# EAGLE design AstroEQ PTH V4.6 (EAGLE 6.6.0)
REVISION: V4.6
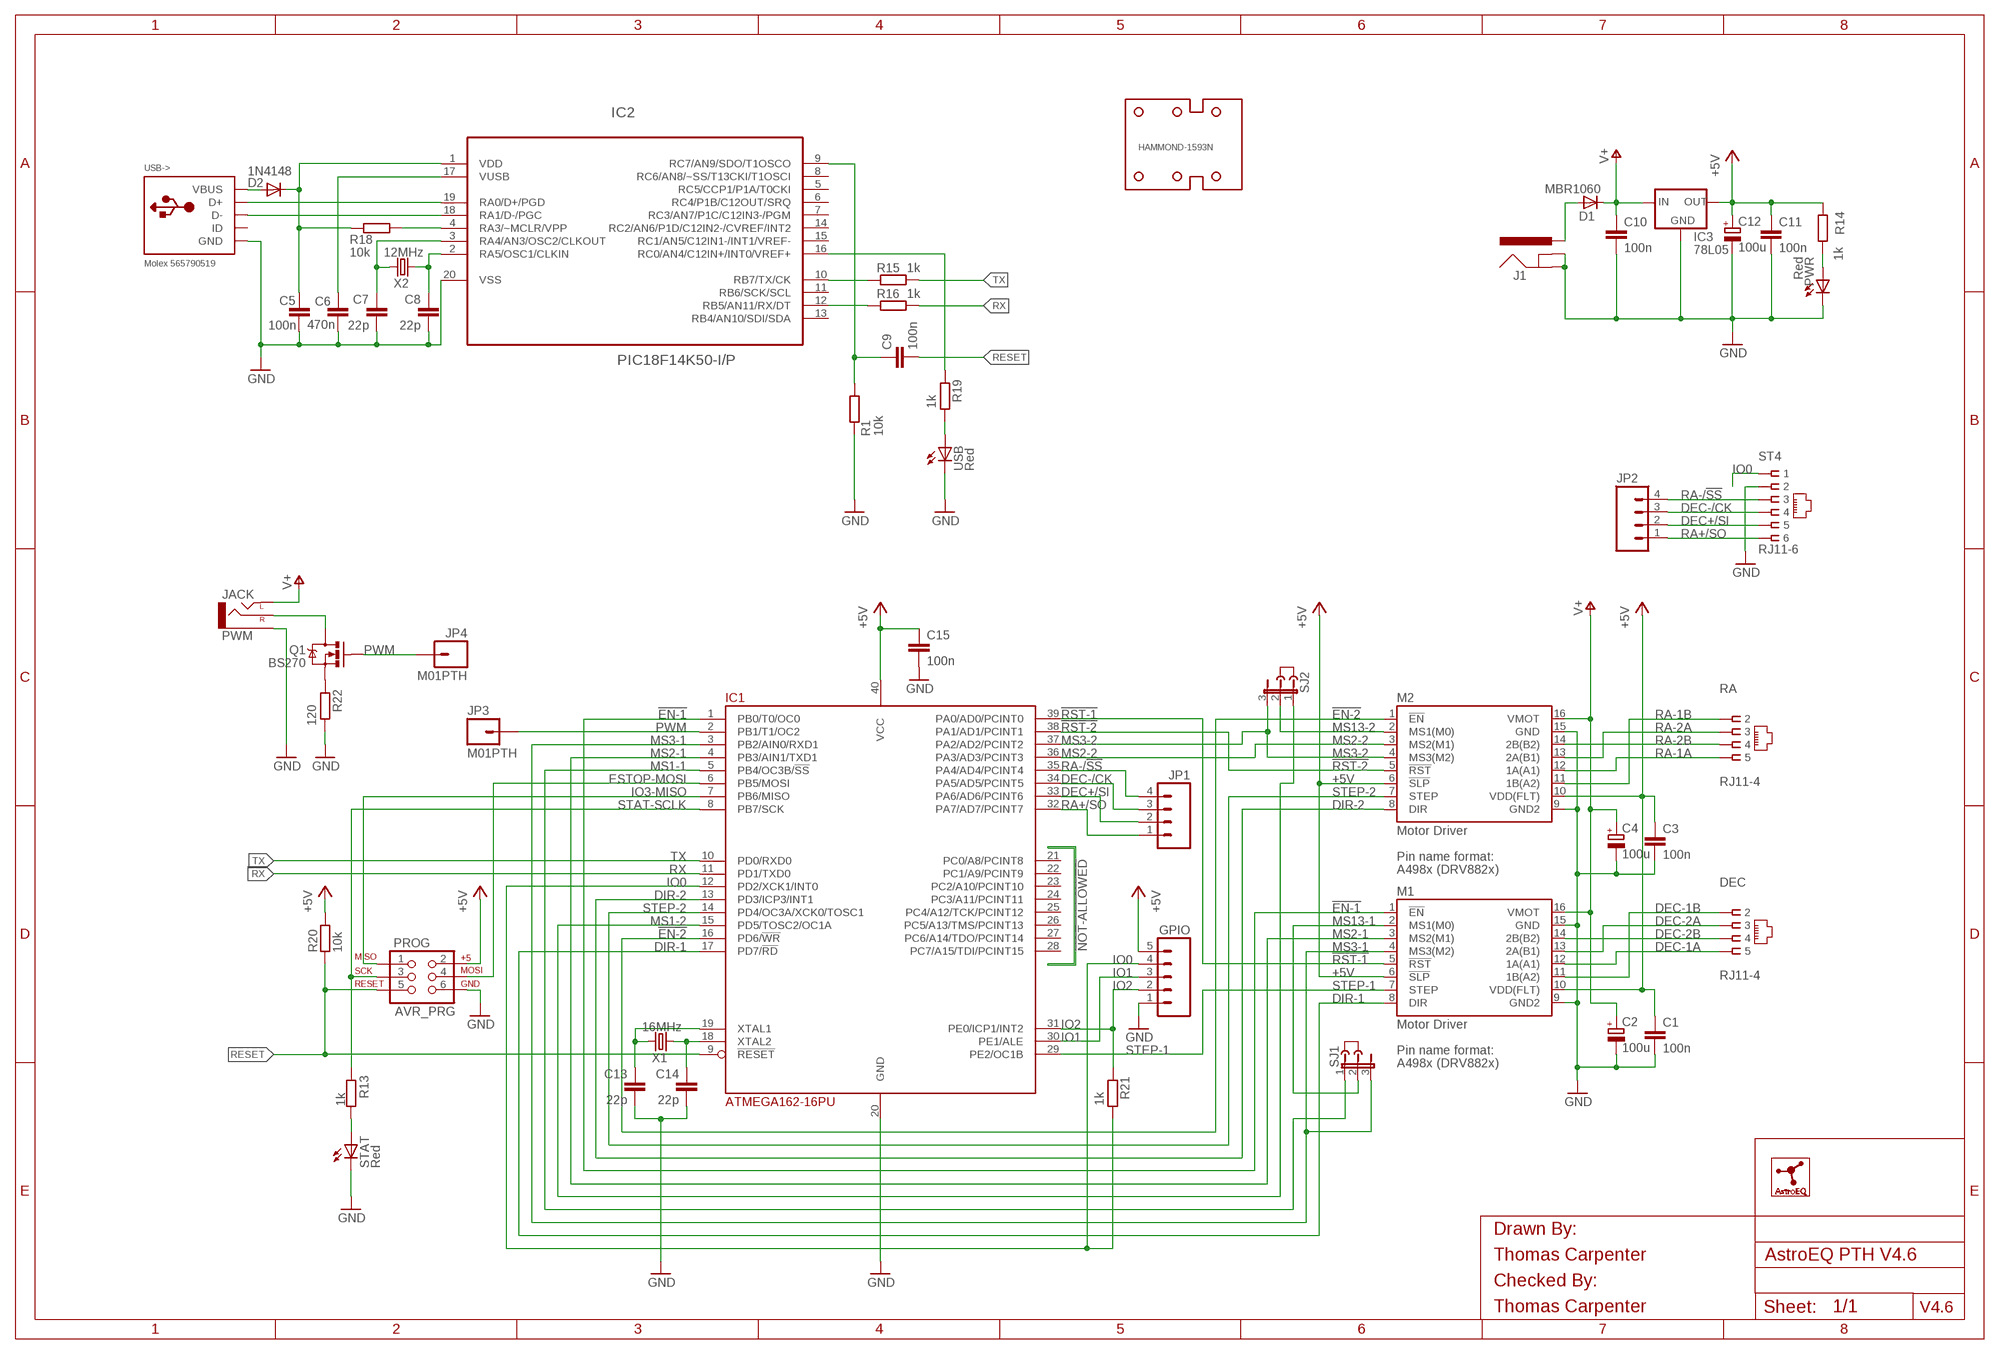
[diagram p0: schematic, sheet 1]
FRAME1 (A3L-LOC): CHECKED_BY: Thomas Carpenter; DRAWN_BY: Thomas Carpenter

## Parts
C1  100n  C-EU025-024X044  [C025-024X044]
C2  100u  CPOL-EUE2.5-7  [E2,5-7]
C3  100n  C-EU025-024X044  [C025-024X044]
C4  100u  CPOL-EUE2.5-7  [E2,5-7]
C5  100n  C-EU025-024X044  [C025-024X044]
C6  470n  C-EU025-024X044  [C025-024X044]
C7  22p  C-EU025-024X044  [C025-024X044]
C8  22p  C-EU025-024X044  [C025-024X044]
C9  100n  C-EU025-024X044  [C025-024X044]
C10  100n  C-EU025-024X044  [C025-024X044]
C11  100n  C-EU025-024X044  [C025-024X044]
C12  100u  CPOL-EUE2.5-7  [E2,5-7]
C13  22p  C-EU025-024X044  [C025-024X044]
C14  22p  C-EU025-024X044  [C025-024X044]
C15  100n  C-EU025-024X044  [C025-024X044]
D1  MBR1060  MUR820  [C221B1A]
D2  1N4148  DIODE1N4148  [DIODE-1N4148]
DEC  RJ11-4  [RJ11-NO_SHIELD-4]
GPIO  M05PTH  [1X05]
HAMMOND-1593N  HAMMOND-1593N-4HOLE  [HAMMOND-1593N4HOLES]
IC1  ATMEGA162-16PU  [DIL40]
IC2  PIC18F14K50-I/P  [DIL20]
IC3  78L05  V_REG_78XXTO-92  [TO-92]
J1  POWER_JACKPTH  [POWER_JACK_PTH]
J2  JUMPER  [JUMP]
J3  JUMPER  [JUMP]
JP1  M04PTH  [1X04]
JP2  M04PTH  [1X04]
JP3  M01PTH  [1X01]
JP4  M01PTH  [1X01]
LOGO1  ASTROEQ5MM  [ASTROEQ-SMALL]
M1  Motor Driver  A4983CARRIER  [DIP16-W]
M2  Motor Driver  A4983CARRIER  [DIP16-W]
PROG  AVR_PRG  AVR_SPI_PRG_6PTH  [2X3]
PWM  JACK  AUDIO-JACKPTH  [AUDIO-JACK]
PWR  Red  LED3MM  [LED3MM]
Q1  BS270  MOSFET-NCHANNELPTH  [TO-92]
R1  10k  R-EU_0204/7  [0204/7]
R13  1k  R-EU_0204/7  [0204/7]
R14  1k  R-EU_0204/7  [0204/7]
R15  1k  R-EU_0204/7  [0204/7]
R16  1k  R-EU_0204/7  [0204/7]
R18  10k  R-EU_0204/7  [0204/7]
R19  1k  R-EU_0204/7  [0204/7]
R20  10k  R-EU_0204/7  [0204/7]
R21  1k  R-EU_0204/7  [0204/7]
R22  120  R-EU_0204/7  [0204/7]
RA  RJ11-4  [RJ11-NO_SHIELD-4]
SJ1  JP2E  [JP2]
SJ2  JP2EL  [JP2L]
ST4  RJ11-6  RJ11-2L-B  [RJ11-NO_SHIELD]
STAT  Red  LED3MM  [LED3MM]
USB  Red  LED3MM  [LED3MM]
USB->  Molex 565790519  USBMOLEX  [USB-MINIB-THM-MOLEX]
X1  16MHz  CRYSTALHC49US  [HC49US]
X2  12MHz  CRYSTALHC49US  [HC49US]

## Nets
!EN-1: IC1.1(PB0/T0/OC0) M1.1(!EN)
!EN-2: IC1.16(PD6/!WR) M2.1(!EN)
!RST-1: IC1.39(PA0/AD0/PCINT0) M1.5(!RST)
!RST-2: IC1.38(PA1/AD1/PCINT1) M2.5(!RST)
+5V: C1.1 C3.1 C11.1 C12.+ C15.1 GPIO.5 IC1.40(VCC) IC3.1(OUT) M1.6(!SLP) M1.10(VDD(FLT)) M2.6(!SLP) M2.10(VDD(FLT)) PROG.2 R14.1 R20.2
AVROSC1: C13.1 IC1.19(XTAL1) X1.2
AVROSC2: C14.1 IC1.18(XTAL2) X1.1
D+: IC2.19(RA0/D+/PGD) USB->.D+
D-: IC2.18(RA1/D-/PGC) USB->.D-
DEC+/SI: IC1.33(PA6/AD6/PCINT6) JP1.2 JP2.2 ST4.5
DEC-1A: DEC.5 M1.12(1A(A1))
DEC-1B: DEC.2 M1.11(1B(A2))
DEC-2A: DEC.3 M1.13(2A(B1))
DEC-2B: DEC.4 M1.14(2B(B2))
DEC-/CK: IC1.34(PA5/AD5/PCINT5) JP1.3 JP2.3 ST4.4
DIR-1: IC1.17(PD7/!RD) M1.8(DIR)
DIR-2: IC1.13(PD3/ICP3/INT1) M2.8(DIR)
DTR: C9.1 IC2.9(RC7/AN9/SDO/T1OSCO) R1.1
ESTOP-MOSI: IC1.6(PB5/MOSI) PROG.4
GND: C1.2 C2.- C3.2 C4.- C5.2 C6.1 C7.2 C8.2 C10.2 C11.2 C12.- C13.2 C14.2 C15.2 GPIO.1 IC1.20(GND) IC2.20(VSS) IC3.2(GND) J1.GND J1.GNDBREAK M1.9(GND2) M1.15(GND) M2.9(GND2) M2.15(GND) PROG.6 PWM.SLEEVE PWR.K(C) R1.2 R22.1 ST4.2 STAT.K(C) USB->.GND USB->.GND1(GND) USB->.GND4(GND) USB.K(C)
IO0: GPIO.4 IC1.12(PD2/XCK1/INT0) R21.1 ST4.1
IO1: GPIO.3 IC1.30(PE1/ALE)
IO2: GPIO.2 IC1.31(PE0/ICP1/INT2) R21.2
IO3-MISO: IC1.7(PB6/MISO) PROG.1
MCLR: IC2.4(RA3/~MCLR/VPP) R18.1
MS1-1: IC1.5(PB4/OC3B/!SS) SJ1.1
MS1-2: IC1.15(PD5/TOSC2/OC1A) SJ2.1
MS2-1: IC1.4(PB3/AIN1/TXD1) M1.3(MS2(M1))
MS2-2: IC1.36(PA3/AD3/PCINT3) M2.3(MS2(M1))
MS3-1: IC1.3(PB2/AIN0/RXD1) M1.4(MS3(M2)) SJ1.3
MS3-2: IC1.37(PA2/AD2/PCINT2) M2.4(MS3(M2)) SJ2.3
MS13-1: M1.2(MS1(M0)) SJ1.2
MS13-2: M2.2(MS1(M0)) SJ2.2
PWM: IC1.2(PB1/T1/OC2) JP3.1 JP4.1 Q1.2(G)
PWM-ILIM: Q1.3(S) R22.2
PWM-OUT: PWM.RING(RIGHT) Q1.1(D)
PWRLED: PWR.A R14.2
RA+/SO: IC1.32(PA7/AD7/PCINT7) JP1.1 JP2.1 ST4.6
RA-1A: M2.12(1A(A1)) RA.5
RA-1B: M2.11(1B(A2)) RA.2
RA-2A: M2.13(2A(B1)) RA.3
RA-2B: M2.14(2B(B2)) RA.4
RA-/!SS: IC1.35(PA4/AD4/PCINT4) JP1.4 JP2.4 ST4.3
RESET: C9.2 IC1.9(!RESET) PROG.5 R20.1
RX: IC1.11(PD1/TXD0) R16.1
RX(USB): IC2.12(RB5/AN11/RX/DT) R16.2
STAT-SCLK: IC1.8(PB7/SCK) PROG.3 R13.1
STATLED: R13.2 STAT.A
STEP-1: IC1.29(PE2/OC1B) M1.7(STEP)
STEP-2: IC1.14(PD4/OC3A/XCK0/TOSC1) M2.7(STEP)
TX: IC1.10(PD0/RXD0) R15.1
TX(USB): IC2.10(RB7/TX/CK) R15.2
USBLED: R19.1 USB.A
USBOSC1: C8.1 IC2.2(RA5/OSC1/CLKIN) X2.1
USBOSC2: C7.1 IC2.3(RA4/AN3/OSC2/CLKOUT) X2.2
USBSTAT: IC2.16(RC0/AN4/C12IN+/INT0/VREF+) R19.2
V+: C2.+ C4.+ C10.1 D1.C IC3.3(IN) M1.16(VMOT) M2.16(VMOT) PWM.TIP(LEFT)
VBUS: D2.A USB->.VBUS
VIN: D1.A J1.PWR
VPIC: C5.1 D2.C IC2.1(VDD) R18.2
VUSB: C6.2 IC2.17(VUSB)
Unconnected: IC1.21(PC0/A8/PCINT8) IC1.22(PC1/A9/PCINT9) IC1.23(PC2/A10/PCINT10) IC1.24(PC3/A11/PCINT11) IC1.25(PC4/A12/TCK/PCINT12) IC1.26(PC5/A13/TMS/PCINT13) IC1.27(PC6/A14/TDO/PCINT14) IC1.28(PC7/A15/TDI/PCINT15) IC2.5(RC5/CCP1/P1A/T0CKI) IC2.6(RC4/P1B/C12OUT/SRQ) IC2.7(RC3/AN7/P1C/C12IN3-/PGM) IC2.8(RC6/AN8/~SS/T13CKI/T1OSCI) IC2.11(RB6/SCK/SCL) IC2.13(RB4/AN10/SDI/SDA) IC2.14(RC2/AN6/P1D/C12IN2-/CVREF/INT2) IC2.15(RC1/AN5/C12IN1-/INT1/VREF-) USB->.ID

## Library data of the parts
C1 C3 C5 C9-C11 C15 = resistor:C-EU: CAPACITOR, European symbol; MF: AVX; MPN: SR205C104KAR; OC_FARNELL: 1100367
C2 C4 C12 = resistor:CPOL-EU: POLARIZED CAPACITOR, European symbol; MF: MULTICOMP; MPN: MCGPR25V107M6.3X11; OC_FARNELL: 9451188
C6 = resistor:C-EU: CAPACITOR, European symbol; MF: KEMET; MPN: C320C474M5U5TA; OC_FARNELL: 1457660
C7 C8 C13 C14 = resistor:C-EU: CAPACITOR, European symbol; MF: AVX; MPN: SR151A220JAR; OC_FARNELL: 1100369
D1 = diode:MUR820: DIODE; MF: MULTICOMP; MPN: MBR1060; OC_FARNELL: 1625119
D2 = SparkFun:DIODE: Diode; MF: MULTICOMP; MPN: 1N4148.; OC_FARNELL: 9565124
DEC RA = con-tycoelectronics:RJ11-4; MF: MOLEX; MPN: 95501-2641; OC_FARNELL: 1560166
GPIO = SparkFun:M05: Header 5 Standard 5-pin 0.1" header. Use with straight break away headers (SKU : PRT-00116), right angle break away headers (PRT-00553), swiss pins (PRT-00743), machine pins (PRT-00117), and female headers (PRT-00115). Molex polarized connector foot print use with SKU : PRT-08230 with associated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; MF: CYNERGY3; MPN: SSF211X050; OC_FARNELL: 4249100
HAMMOND-1593N = holes:HAMMOND-1593N; MF: HAMMOND; MPN: 1593NBK; OC_FARNELL: 9287566
IC1 = atmel:ATMEGA162: 8-bit RISC MICROCONTROLLER 16K Bytes internal flash program memory 1K Bytes internal SRAM Upto 64K Bytes optional external memory space 512 Bytes EEPROM Two 8-bit timers Two 16-bit timers Dual programmable serial USARTs Master/Slave serial SPI interface Source: ATMEGA162_DIP40.lbr; MF: ATMEL; MPN: ATMEGA162-16PU; OC_FARNELL: 9171169
IC2 = microchip:PIC18F14K50-I/P: USB Flash Microcontrollers; MF: MICROCHIP; MPN: PIC18F14K50-I/P; OC_FARNELL: 1648501; OC_NEWARK: 77M3103; PACKAGE: DIP-20; SUPPLIER: Microchip
IC3 = SparkFun:V_REG_78XX: Voltage Regulator Standard 7805 5V regulator. IGO (Input Ground Output). Spark Fun Electronics SKU : COM-00107; MF: FAIRCHILD SEMICONDUCTOR; MPN: LM78L05ACZX; OC_FARNELL: 1467367
J1 = SparkFun:POWER_JACK: Power Jack This is the standard 5.5mm barrel jack for power. The PTH is the most common, proven, reliable, footprint. All others are experimental. The Slot footprint only works if the mill layer is transmitted to the PCB fab house so be warned. Spark Fun Electronics SKU : PRT-00119. Mating wall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; MF: MULTICOMP; MPN: MJ-179PH; OC_FARNELL: 1737246
J2 J3 = jumper:JUMPER: JUMPER header; OC_FARNELL: unknown
JP1 JP2 = SparkFun:M04: Header 4 Standard 4-pin 0.1" header. Use with straight break away headers (SKU : PRT-00116), right angle break away headers (PRT-00553), swiss pins (PRT-00743), machine pins (PRT-00117), and female headers (PRT-00115). Molex polarized connector foot print use with SKU : PRT-08231 with associated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; OC_FARNELL: unknown
JP3 JP4 = SparkFun:M01: Header 1; OC_FARNELL: unknown
LOGO1 = CompanyLogos:ASTROEQ; OC_FARNELL: unknown
M1 M2 = A4983Carrier:A4983CARRIER; MF: SAMTEC; MPN: CES-116-01-T-S; OC_FARNELL: 1667522
PROG = SparkFun:AVR_SPI_PRG_6: AVR ISP 6 Pin This is the reduced ISP connector for AVR programming. Common on Arduino. This footprint will take up less PCB space and can be used with a 10-pin to 6-pin adapter such as SKU: BOB-08508; MF: TE CONNECTIVITY / AMP; MPN: 826632-3; OC_FARNELL: 3418492
PWM = SparkFun:AUDIO-JACK: 3.5mm Audio Jack Simple 3.5mm common PCB mount audio jack. SKU: PRT-08032; MF: CLIFF ELECTRONIC COMPONENTS; MPN: FC68131; OC_FARNELL: 2518188
PWR STAT USB = led:LED: LED; MF: KINGBRIGHT; MPN: L-424HDT; OC_FARNELL: 1142499
Q1 = SparkFun:MOSFET-NCHANNEL; MF: FAIRCHILD SEMICONDUCTOR; MPN: BS270; OC_FARNELL: 1017689
R1 R18 R20 = rcl:R-EU_: RESISTOR, European symbol; MF: MULTICOMP; MPN: MF12 10K; OC_FARNELL: 9342419
R13-R16 R19 R21 = rcl:R-EU_: RESISTOR, European symbol; MF: MULTICOMP; MPN: MF12 1K; OC_FARNELL: 9342400
R22 = rcl:R-EU_: RESISTOR, European symbol; MF: MULTICOMP; MPN: MF12 120R; OC_FARNELL: 9342516
SJ1 SJ2 = jumper:JP2E: JUMPER; OC_FARNELL: unknown
ST4 = con-tycoelectronics:RJ11: CORCOM Modular RJ Jacks No Shield Source: www.tycoelectronics.com .. ENG_DS_1654001_1099_RJ_L_0507.pdf; MF: MOLEX; MPN: 95501-2661; OC_FARNELL: 1536490; OC_NEWARK: 83F4463
USB-> = adafruit:USB: USB Connectors USBMINIB - Surface Mount Female Mini-B USB Connector 4UConnector: 06564 By microbuilder.eu Thru-hole RA Female Mini-B USB Connector 4UConnector: 18732 By ladyada.net; MF: MOLEX; MPN: 565790519; OC_FARNELL: 1125347
X1 = SparkFun:CRYSTAL: Crystals; MF: TXC; MPN: 9B-16.000MEEJ-B; OC_FARNELL: 1842217
X2 = SparkFun:CRYSTAL: Crystals; MF: TXC; MPN: 9B-12.000MAAJ-B; OC_FARNELL: 1842203

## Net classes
1 power: width 0.61 mm, drill 0.711 mm, clearance 0.203 mm
2 gnd: width 0.305 mm, drill 0.711 mm, clearance 0.203 mm
3 usbvcc: width 0.508 mm, drill 0.711 mm, clearance 0.203 mm

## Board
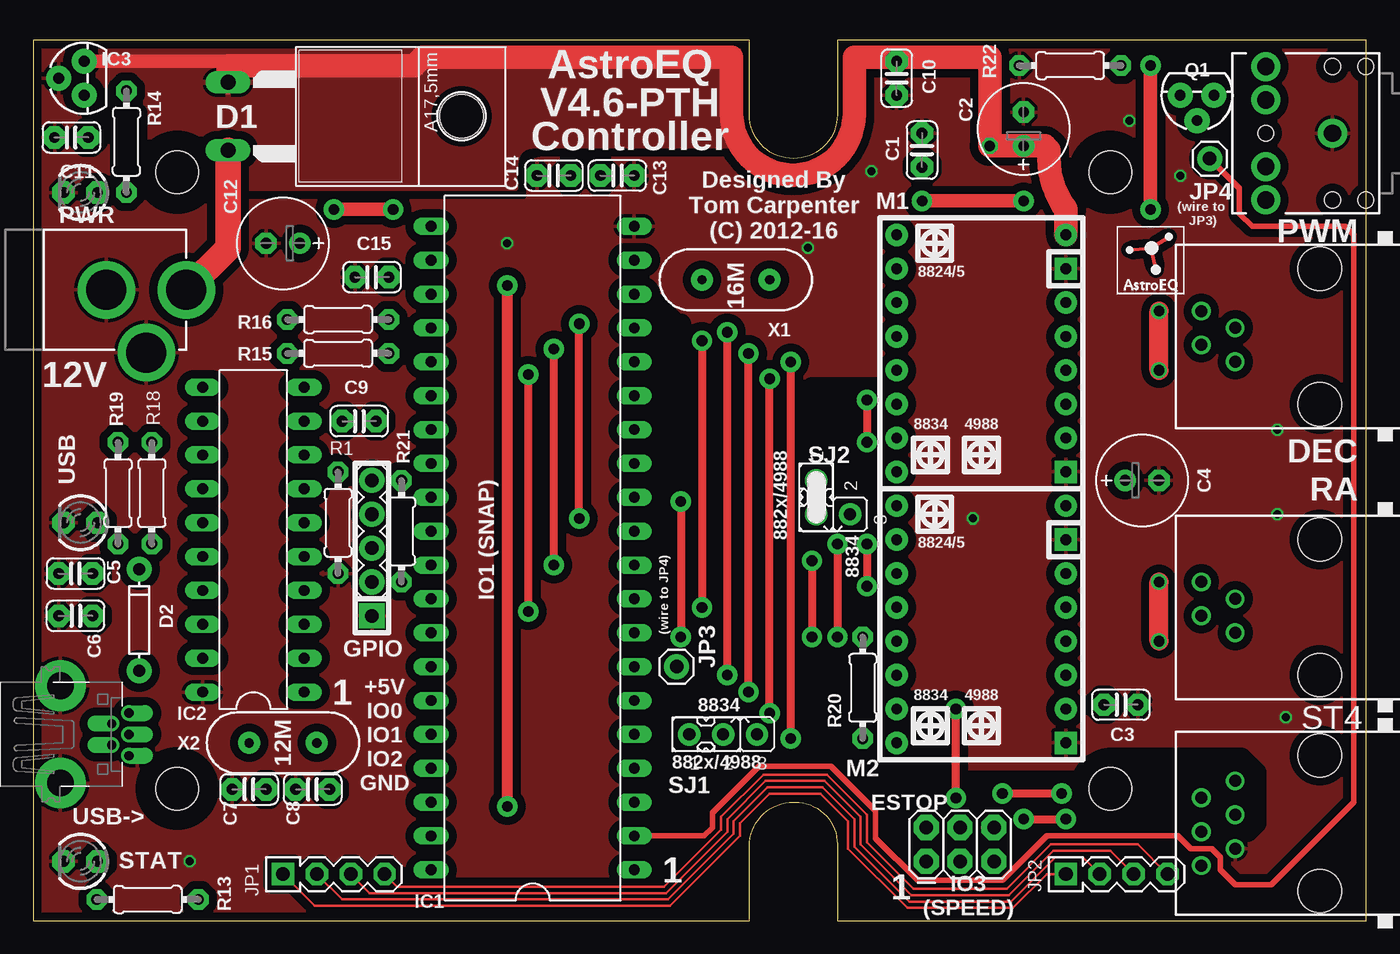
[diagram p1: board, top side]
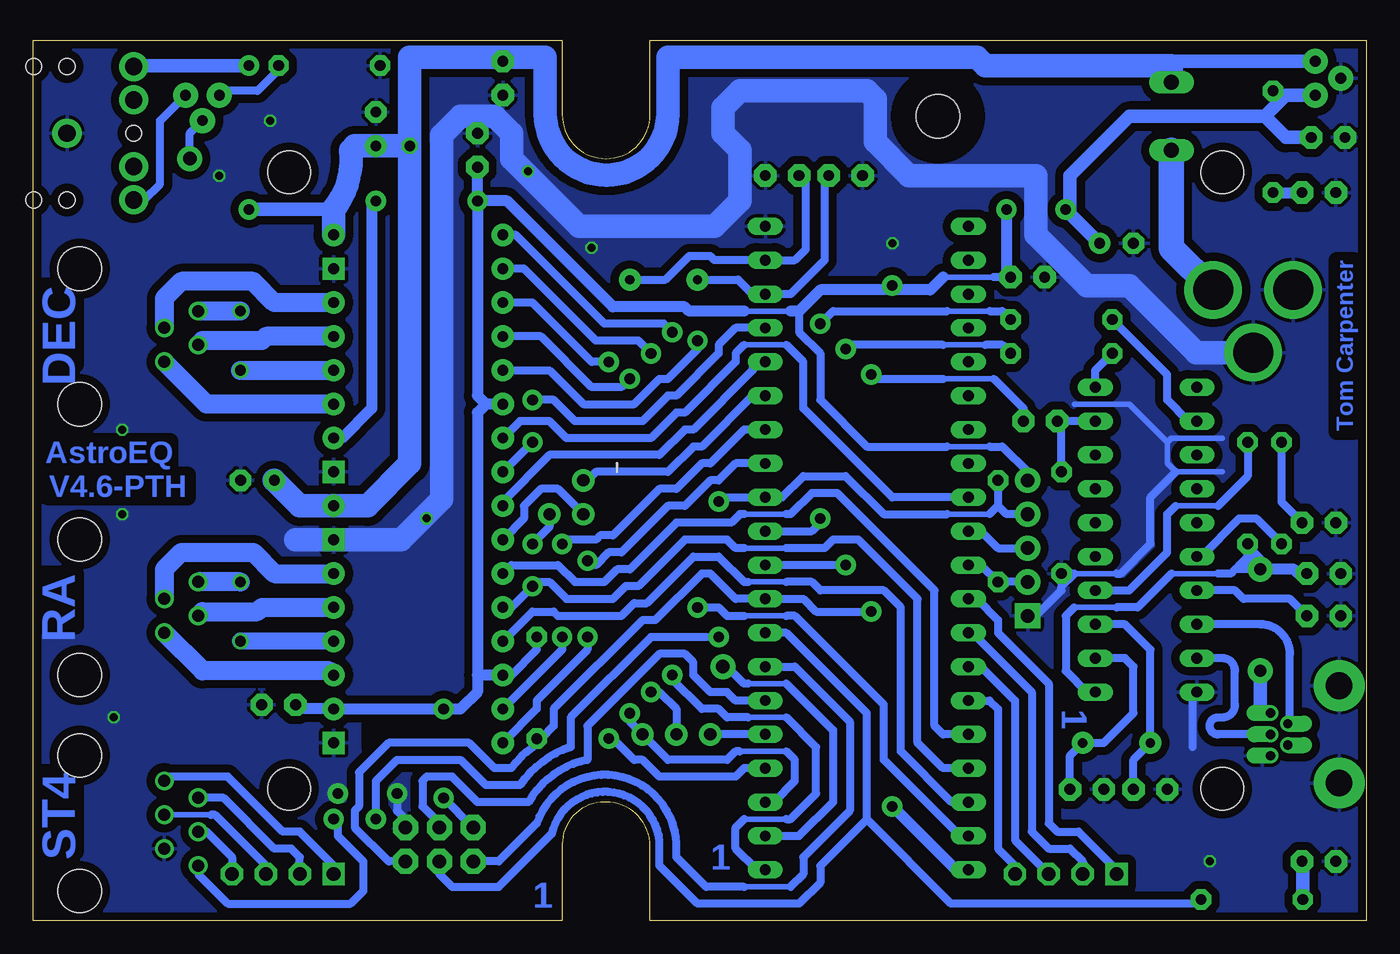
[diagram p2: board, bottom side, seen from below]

Size 100 x 66.04 mm. Coordinates in mm from the lower left corner, seen from the top.
Outline: 57.02,8.89 57.15,8.89
Copper layers (1*16): Top 0.035mm / dielectric 1.5mm / Bottom 0.035mm
Design rules "default *": minimum track width 6mil, minimum drill 12mil, track to track 6mil, track to pad 6mil, pad to pad 6mil, via to via 6mil, smd to smd 0mil, copper to edge 10mil, drill to drill 10mil, minimum pad ring 10mil, minimum via ring 6mil, stop-mask expansion 2mil, vias tented up to drill 1mm, thermal gap 10mil
tKeepout: area 78.3,7.4 to 83.3,12.4; area 78.3,53.6 to 83.3,58.6; area 8.3,7.4 to 13.3,12.4; area 8.3,53.6 to 13.3,58.6
bKeepout: area 78.3,7.4 to 83.3,12.4; area 78.3,53.6 to 83.3,58.6; area 8.3,7.4 to 13.3,12.4; area 8.3,53.6 to 13.3,58.6
tRestrict: area 78.3,53.6 to 83.3,58.6; area 8.3,7.4 to 13.3,12.4; area 8.3,53.6 to 13.3,58.6; area 6.3,56.2 to 7.9,60.6; 34 lines
bRestrict: 1 lines

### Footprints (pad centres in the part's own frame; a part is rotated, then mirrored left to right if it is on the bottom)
C025-024X044 = drill 0.813 pad 1.676 octagon: 1 -1.27,0; 2 1.27,0
E2,5-7 = drill 0.813 pad 1.6: + -1.27,0 | drill 0.813 pad 1.6 octagon: - 1.27,0
C221B1A = drill 1.118 long: A 2.54,-6.35; C -2.54,-6.35 | hole 3.302: 0,11.176
DIODE-1N4148 = drill 0.9 pad 1.88: A -3.81,0; C 3.81,0
RJ11-NO_SHIELD-4 = drill 0.9 pad 1.4: 2 -1.905,6.35; 3 -0.635,8.89; 4 0.635,6.35; 5 1.905,8.89 | hole 3.251: -5.08,0; 5.08,0
1X05 = drill 1.016 pad 1.88 square: 1 -5.08,0 | drill 1.016 pad 1.88: 2 -2.54,0; 3 0,0; 4 2.54,0; 5 5.08,0
HAMMOND-1593N4HOLES = hole 3.2: 10.795,9.906; 10.795,56.134; 80.797,9.906; 80.797,56.134
DIL40 = drill 0.813 long: 1 -24.13,-7.62; 2 -21.59,-7.62; 3 -19.05,-7.62; 4 -16.51,-7.62; 5 -13.97,-7.62; 6 -11.43,-7.62; 7 -8.89,-7.62; 8 -6.35,-7.62; 9 -3.81,-7.62; 10 -1.27,-7.62; 11 1.27,-7.62; 12 3.81,-7.62; 13 6.35,-7.62; 14 8.89,-7.62; 15 11.43,-7.62; 16 13.97,-7.62; 17 16.51,-7.62; 18 19.05,-7.62; 19 21.59,-7.62; 20 24.13,-7.62; 21 24.13,7.62; 22 21.59,7.62; 23 19.05,7.62; 24 16.51,7.62; 25 13.97,7.62; 26 11.43,7.62; 27 8.89,7.62; 28 6.35,7.62; 29 3.81,7.62; 30 1.27,7.62; 31 -1.27,7.62; 32 -3.81,7.62; 33 -6.35,7.62; 34 -8.89,7.62; 35 -11.43,7.62; 36 -13.97,7.62; 37 -16.51,7.62; 38 -19.05,7.62; 39 -21.59,7.62; 40 -24.13,7.62
DIL20 = drill 0.813 long: 1 -3.81,11.43; 2 -3.81,8.89; 3 -3.81,6.35; 4 -3.81,3.81; 5 -3.81,1.27; 6 -3.81,-1.27; 7 -3.81,-3.81; 8 -3.81,-6.35; 9 -3.81,-8.89; 10 -3.81,-11.43; 11 3.81,-11.43; 12 3.81,-8.89; 13 3.81,-6.35; 14 3.81,-3.81; 15 3.81,-1.27; 16 3.81,1.27; 17 3.81,3.81; 18 3.81,6.35; 19 3.81,8.89; 20 3.81,11.43
TO-92 = drill 0.813 pad 1.88: 1 -1.27,0; 2 0,1.905; 3 1.27,0
POWER_JACK_PTH = drill 2.997 pad 4.318: GND 0,7.7; GNDBREAK 4.7,10.7; PWR 0,13.7
1X04 = drill 1.016 pad 1.676 square: 1 0,0 | drill 1.016 pad 1.676 octagon: 2 2.54,0; 3 5.08,0; 4 7.62,0
1X01 = drill 1.016 pad 1.88: 1 0,0
DIP16-W = drill 0.813 pad 1.676: 1 -8.89,-6.35; 2 -6.35,-6.35; 3 -3.81,-6.35; 4 -1.27,-6.35; 5 1.27,-6.35; 6 3.81,-6.35; 7 6.35,-6.35; 8 8.89,-6.35; 10 6.35,6.35; 11 3.81,6.35; 12 1.27,6.35; 13 -1.27,6.35; 14 -3.81,6.35; 16 -8.89,6.35 | drill 0.813 pad 1.676 square: 9 8.89,6.35; 15 -6.35,6.35
2X3 = drill 1.016 pad 1.88 octagon: 1 -2.54,-1.27; 2 -2.54,1.27; 3 0,-1.27; 4 0,1.27; 5 2.54,-1.27; 6 2.54,1.27
AUDIO-JACK = drill 1.3 pad 2.184: RING 5,5; RSH 5,2.5; SLEEVE 0,0; TIP 5,-5; TSH 5,-2.5 | hole 1.2: 0,5; -2.5,5; -2.5,-5; 0,-5; 5,0
LED3MM = drill 0.813 pad 1.676 octagon: A -1.27,0; K 1.27,0
0204/7 = drill 0.813 pad 1.524 octagon: 1 -3.81,0; 2 3.81,0
JP2 = drill 0.914 pad 1.676: 1 -2.54,0; 2 0,0; 3 2.54,0
JP2L = drill 0.914 pad 1.676: 1 -2.54,0; 2 0,0; 3 0,2.54
RJ11-NO_SHIELD = drill 0.9 pad 1.4: 1 -3.175,8.89; 2 -1.905,6.35; 3 -0.635,8.89; 4 0.635,6.35; 5 1.905,8.89; 6 3.175,6.35 | hole 3.251: -5.08,0; 5.08,0
USB-MINIB-THM-MOLEX = drill 0.7 offset: D+ 0,9.72; D- -0.8,8.42; GND 1.6,9.72; ID 0.8,8.42; VBUS -1.6,9.72 | drill 2 pad 3.81: GND1 -3.65,4.57; GND4 3.65,4.57
HC49US = drill 0.7 pad 1.651: 1 -2.54,0; 2 2.54,0

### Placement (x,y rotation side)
C1  66.67,57.78 90 top
C2  74.3,59.37 90 top
C3  81.6,16.19 0 top
C4  83.19,33.02 0 top
C5  3.17,26.04 180 top
C6  3.17,22.86 0 top
C7  16.19,9.84 180 top
C8  20.95,9.84 180 top
C9  24.45,37.47 0 top
C10  64.77,63.18 270 top
C11  2.86,58.74 180 top
C12  18.73,50.8 180 top
C13  43.81,55.88 0 top
C14  39.05,55.88 180 top
C15  25.4,48.26 180 top
D1  20.95,60.33 270 top
D2  7.94,22.54 90 top
DEC  96.52,43.81 90 top
GPIO  25.4,27.94 90 top
HAMMOND-1593N  0,0 0 top
IC1  37.47,27.94 90 top
IC2  16.51,28.57 180 top
IC3  3.81,63.18 90 top
J1  -2.22,47.31 270 top
J2  58.74,31.75 0 top
J3  50.48,13.97 90 top
JP1  18.73,3.49 0 top
JP2  77.47,3.49 0 top
JP3  48.26,19.05 0 top
JP4  88.27,57.15 0 top
LOGO1  81.28,46.99 0 top
M1  71.12,42.55 270 top
M2  71.12,22.23 270 top
PROG  69.53,5.71 0 top
PWM  97.47,59.05 180 top
PWR  3.54,54.61 180 top
Q1  87.31,61.91 180 top
R1  22.86,29.84 270 top
R13  8.57,1.59 180 top
R14  6.99,58.42 270 top
R15  22.86,42.55 180 top
R16  22.86,45.09 180 top
R18  8.89,32.07 270 top
R19  6.35,32.07 270 top
R20  62.23,17.46 90 top
R21  27.62,29.21 270 top
R22  77.79,64.14 0 top
RA  96.52,23.5 90 top
SJ1  51.75,13.97 0 top
SJ2  58.74,30.48 270 top
ST4  96.52,7.3 90 top
STAT  3.54,4.45 180 top
USB  3.54,29.84 180 top
USB->  -2.54,13.97 270 top
X1  52.7,48.07 0 top
X2  18.73,13.34 180 top

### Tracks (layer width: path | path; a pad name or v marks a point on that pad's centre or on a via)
!EN-1  (via drill 0.8 pad 1.52)
  Top 0.61: v52.07,18.41 v52.07,44.13
  Bottom 0.406: 46.67,7.62 43.5,7.62 | 43.5,15.24 46.35,15.24
  Bottom 0.61: IC1.1 45.72,3.81 47.31,5.4 47.31,6.99 46.67,7.62 | 43.5,7.62 43.18,7.62 41.27,9.53 41.27,13.02 43.5,15.24 | 46.35,15.24 47.94,15.24 48.58,15.88 49.85,15.88 52.07,18.1 v52.07,18.41 | v52.07,44.13 52.7,44.77 57.15,44.77 63.82,51.44 M1.1
!EN-2
  Bottom 0.61: IC1.16 46.04,41.91 46.04,41.27 50.48,36.83 51.12,36.83 53.02,34.92 61.28,34.92 64.77,31.43 M2.1
!RST-1  (via drill 0.8 pad 1.52)
  Top 0.61: v50.16,43.5 v50.16,23.5
  Bottom 0.406: 43.5,22.86 46.67,22.86
  Bottom 0.61: IC1.39 30.48,6.35 36.2,12.06 36.2,16.19 42.86,22.86 43.5,22.86 | M1.5 61.28,41.27 58.74,38.73 54.93,38.73 53.02,40.64 52.39,40.64 50.16,42.86 v50.16,43.5 | v50.16,23.5 48.58,23.5 47.94,22.86 46.67,22.86
!RST-2
  Bottom 0.406: 43.5,25.4 46.35,25.4
  Bottom 0.61: IC1.38 31.11,8.89 34.92,12.7 34.92,23.5 36.2,24.77 40.96,24.77 41.59,25.4 43.5,25.4 | M2.5 62.55,23.18 60.96,23.18 60.64,22.86 55.88,22.86 54.93,23.81 53.98,23.81 50.48,27.3 48.58,27.3 46.67,25.4 46.35,25.4
+5V  (via drill 0.8 pad 1.52)
  Top 0.61: v69.22,9.21 v69.22,15.88
  Top 0.813: v35.56,47.62 v35.56,8.57
  Top 1.016: v66.67,53.98 v74.3,53.98 | v22.54,53.34 v26.99,53.34
  Bottom 0.406: 27.94,48.26 31.75,48.26 | 43.18,45.72 46.67,45.72 | 31.43,35.56 28.26,35.56
  Bottom 0.61: 26.99,48.26 27.94,48.26 | PROG.2 v69.22,9.21 | v35.56,47.62 35.56,47.31 | IC1.40 30.8,3.81 | 67.94,15.88 v69.22,15.88 | M2.6 64.14,18.41 62.23,20.32 R20.2 | 42.55,45.72 42.55,44.13 40.96,42.55 40.96,39.05 37.47,35.56 31.43,35.56 | 28.26,35.56 27.3,35.56 25.4,33.66 GPIO.5
  Bottom 0.813: v66.67,53.98 C1.1 | C15.1 26.99,48.26 v26.99,53.34 | 31.75,48.26 32.7,47.31 35.56,47.31 40.96,47.31 42.55,45.72 43.18,45.72 | 46.67,45.72 50.8,45.72 51.12,46.04 56.52,46.04 64.45,53.98 v66.67,53.98 | 22.23,53.66 22.23,53.34 v22.54,53.34 | 30.8,3.81 v35.56,8.57 | v66.67,53.98 66.67,39.37 66.04,38.73 | 66.04,38.73 66.67,38.1 66.67,18.41 | 66.67,18.41 66.67,17.14 67.94,15.88 M2.10 80.01,15.88 C3.1 | M2.6 66.67,18.41 | M1.6 66.04,38.73 | v74.3,53.98 74.61,53.66 74.61,38.42 76.83,36.2 M1.10
  Bottom 1.016: IC3.1 6.03,61.91 6.35,61.59 | 6.35,61.59 7.62,60.33 | 7.62,60.33 17.78,60.33 22.23,55.88 22.23,53.66 22.23,53.02 C12.+ | R14.1 6.35,61.59 | C11.1 6.03,58.74 7.62,60.33
AVROSC1
  Bottom 0.61: C13.1 42.07,55.4 42.07,50.32 42.86,49.53 IC1.19 48.9,49.53 49.21,49.85 50.8,49.85 52.58,48.07 X1.2
AVROSC2
  Bottom 0.61: C14.1 40.64,55.56 40.64,49.53 43.18,46.99 IC1.18 46.04,46.99 47.12,48.07 X1.1
D+
  Bottom 0.61: USB->.D+ 11.11,13.97 arc90 11.75,14.61 arc90 11.11,15.24 10.79,15.24 arc-90 9.84,16.19 9.84,18.73 arc-90 10.79,19.68 IC2.19
D-
  Bottom 0.61: USB->.D- 5.71,14.77 5.71,20 arc-90 7.94,22.23 IC2.18
DEC+/SI
  Top 0.203: JP1.2 23.18,1.59 47.62,1.59 52.55,6.51 52.55,7.46 55.09,10 59.21,10 61.59,7.62 61.59,5.56 65.72,1.43 73.34,1.43 76.68,4.76 78.74,4.76 JP2.2
  Bottom 0.61: IC1.33 29.53,21.59 25.08,17.14 25.08,6.67 23.81,5.4 22.23,5.4 21.27,4.45 JP1.2 | JP2.2 80.01,4.76 80.64,5.4 81.92,5.4 85.72,9.21 ST4.5
DEC-1A  (via drill 0.8)
  Top 1.422: v84.45,41.27 v84.45,45.72
  Bottom 1.422: v84.45,45.72 DEC.5 | v84.45,41.27 M1.12
DEC-1B
  Bottom 1.422: M1.11 87,38.73 DEC.2
DEC-2A
  Bottom 1.422: M1.13 82.55,43.81 82.87,43.5 87.31,43.5 DEC.3
DEC-2B
  Bottom 1.422: M1.14 81.92,46.35 83.5,47.94 88.9,47.94 90.17,46.67 DEC.4
DEC-/CK
  Top 0.203: JP1.3 25.24,2.06 47.47,2.06 52.07,6.67 52.07,7.62 54.93,10.48 59.37,10.48 62.07,7.78 62.07,5.71 65.88,1.91 73.18,1.91 76.52,5.24 80.8,5.24 JP2.3
  Bottom 0.406: 86.68,7.94 ST4.4
  Bottom 0.61: IC1.34 28.89,19.05 26.35,16.51 26.35,6.03 JP1.3 | 86.68,7.94 86.36,7.94 82.55,4.13 JP2.3
DIR-1  (via drill 0.8 pad 1.52)
  Top 0.61: v62.55,39.05 v62.55,35.88
  Bottom 0.61: IC1.17 47.31,44.45 48.58,43.18 48.58,42.55 51.75,39.37 52.39,39.37 54.29,37.47 59.37,37.47 60.96,39.05 v62.55,39.05 | v62.55,35.88 M1.8
DIR-2  (via drill 0.8 pad 1.52)
  Top 0.61: v58.42,26.99 v58.42,21.27
  Bottom 0.61: IC1.13 47.31,34.29 48.58,33.02 49.21,33.02 51.12,31.11 52.39,31.11 55.88,27.62 56.83,27.62 57.78,26.67 58.1,26.67 v58.42,26.99 | v58.42,21.27 58.42,20.32 62.23,16.51 62.23,15.88 M2.8
DTR
  Bottom 0.61: IC2.9 C9.1 22.86,37.47 R1.1
ESTOP-MOSI
  Bottom 0.61: IC1.6 47.31,16.51 47.94,17.14 49.21,17.14 50.48,18.41 50.48,19.37 51.12,20 53.02,20 58.42,14.61 58.42,12.06 arc-48 62.85,8.89 66.67,8.89 68.58,10.79 70.48,10.79 70.8,10.48 70.8,8.57 69.53,7.3 PROG.4
GND  (via drill 0.6, 0.8 pad 1.52)
  Top 0.61: v77.15,9.53 v72.71,9.53
  Bottom 0.406: 21.91,26.04 18.73,26.04 | 10.79,33.66 14.29,33.66 14.92,34.29 14.92,35.88 | 14.92,35.88 14.61,36.2 10.79,36.2 | 14.92,35.88 17.78,38.73 21.91,38.73
  Bottom 0.61: 13.02,13.02 13.02,16.83 IC2.20 | GPIO.1 24.77,22.86 22.86,24.77 22.86,25.08 | 22.86,25.08 21.91,26.04 R1.2 22.86,25.08 | 18.73,26.04 18.41,26.04 16.19,28.26 16.19,31.75 14.29,33.66 | v72.71,9.53 72.71,8.26 72.07,7.62 PROG.6
  Bottom 1.778: J1.GNDBREAK 12.76,42.61 17.78,47.62 20.95,47.62 24.77,51.44 24.77,55.88 34.29,55.88 36.83,58.42 36.83,61.59 37.47,62.23 46.99,62.23 48.26,60.96 48.26,59.05 46.99,57.78 46.99,53.98 48.9,52.07 59.05,52.07 64.14,57.15 64.14,59.05 65.41,60.33 67.94,60.33 69.37,58.9 69.37,31.59 72.39,28.57 80.33,28.57
  other vias: 35.56,50.8 93.98,15.24 82.23,60.01 93.34,36.83 70.48,30.16 62.87,56.2 11.75,4.45 58.1,50.48 86.04,55.88 93.34,30.48
  pour Top (isolate 0.61, rank 2): -1.27,66.99 101.03,66.99 101.03,-0.95 -1.27,-0.95
  pour Bottom (isolate 0.61): -1.27,66.99 101.03,66.99 101.03,-0.95 -1.27,-0.95
IO0  (via drill 0.8 pad 1.52)
  Top 0.61: v48.58,31.43 v48.58,21.27 | v74.3,7.62 v77.47,7.62
  Bottom 0.406: 31.43,30.48 28.26,30.48
  Bottom 0.61: 31.43,30.48 36.2,30.48 39.05,33.34 42.23,33.34 43.81,31.75 IC1.12 47.94,31.75 48.26,31.43 v48.58,31.43 | R21.1 27.62,31.11 | 27.62,31.11 28.26,30.48 | 27.62,31.11 26.99,30.48 GPIO.4 | v48.58,21.27 53.66,21.27 59.69,15.24 59.69,13.02 arc-37 63.5,10.16 66.04,10.16 67.94,12.06 72.71,12.06 74.3,10.48 v74.3,7.62 | ST4.1 87.63,3.49 85.41,1.27 76.2,1.27 75.25,2.22 75.25,4.45 77.15,6.35 77.15,7.62 v77.47,7.62
IO1
  Bottom 0.61: IC1.30 28.89,29.21 27.62,27.94 GPIO.3
IO2
  Bottom 0.61: IC1.31 28.89,26.67 R21.2 GPIO.2
IO3-MISO
  Bottom 0.406: 43.18,2.54 46.67,2.54
  Bottom 0.61: IC1.7 42.86,19.05 38.73,14.92 38.73,8.26 42.23,4.76 42.23,3.49 43.18,2.54 | 46.67,2.54 49.53,2.54 51.75,4.76 51.75,5.71 arc-159 62.23,7.3 65.09,4.45 PROG.1
MCLR
  Bottom 0.406: 14.29,31.11 11.11,31.11
  Bottom 0.61: IC2.4 17.78,24.77 14.92,27.62 14.92,30.48 14.29,31.11 | 11.11,31.11 8.89,33.34 R18.1
MS1-1
  Bottom 0.61: IC1.5 SJ1.1
MS1-2
  Bottom 0.61: IC1.15 46.04,39.37 49.85,35.56 50.48,35.56 52.39,33.66 57.78,33.66 58.42,33.02 SJ2.1
MS2-1  (via drill 0.8 pad 1.52)
  Top 0.61: v56.83,13.65 v56.83,41.91
  Bottom 0.61: IC1.4 46.67,11.43 47.31,10.79 53.02,10.79 54.29,12.06 54.93,12.06 56.52,13.65 v56.83,13.65 | v56.83,41.91 58.1,41.91 62.55,46.35 M1.3
MS2-2
  Bottom 0.406: 43.5,30.48 46.67,30.48
  Bottom 0.61: IC1.36 31.75,13.97 32.38,14.61 32.38,24.77 39.69,32.07 41.59,32.07 43.18,30.48 43.5,30.48 | 46.67,30.48 46.99,30.48 47.62,29.84 51.75,29.84 55.24,26.35 56.2,26.35 57.15,25.4 59.37,25.4 60.64,26.67 64.14,26.67 M2.3
MS3-1  (via drill 0.8 pad 1.52)
  Top 0.61: v55.24,15.56 v55.24,40.64
  Bottom 0.406: 43.5,12.7 46.99,12.7
  Bottom 0.61: v55.24,40.64 55.88,40.01 58.1,40.01 61.91,43.81 M1.4 | IC1.3 44.45,8.89 42.86,10.48 42.86,12.06 43.5,12.7 | 46.99,12.7 47.31,12.7 47.94,12.06 52.39,12.06 SJ1.3 55.24,14.92 v55.24,15.56
MS3-2  (via drill 0.8 pad 1.52)
  Top 0.61: v62.55,28.26 v62.55,25.08
  Bottom 0.406: 43.5,27.94 46.67,27.94
  Bottom 0.61: IC1.37 31.75,11.43 33.66,13.34 33.66,24.13 38.1,28.57 40.01,28.57 40.64,27.94 43.5,27.94 | 46.67,27.94 47.31,27.94 47.94,28.57 51.12,28.57 54.61,25.08 55.56,25.08 56.52,24.13 60.01,24.13 61.28,25.4 62.23,25.4 v62.55,25.08 64.14,23.5 M2.4 | SJ2.3 61.28,29.53 v62.55,28.26
MS13-1  (via drill 0.8 pad 1.52)
  Top 0.61: v53.66,17.14 v53.66,42.55
  Bottom 0.61: v53.66,42.55 54.61,43.5 57.78,43.5 63.18,48.9 M1.2 | v53.66,17.14 53.02,17.14 51.75,15.88 SJ1.2
MS13-2
  Bottom 0.61: 65.09,28.57 M2.2 63.18,30.16 63.18,31.11 61.91,32.38 60.64,32.38 SJ2.2
PWM
  Top 0.406: IC1.2 50.32,6.35 50.96,6.99 50.96,8.1 54.45,11.59 59.85,11.59 63.18,8.26 63.18,6.19 66.36,3.02 72.71,3.02 76.04,6.35 85.88,6.35 86.84,5.4 88.42,5.4 89.06,4.76 89.06,3.81 90.17,2.7 92.87,2.7 99.06,8.89 99.06,51.44 98.42,52.07 91.44,52.07 90.49,53.02 90.49,54.93 JP4.1
  Bottom 0.406: 43.5,17.78 46.35,17.78
  Bottom 0.61: 46.35,17.78 46.67,17.78 47.94,19.05 JP3.1 | 43.5,17.78 40.01,14.29 40.01,8.89 42.55,6.35 IC1.2 | JP4.1 88.27,59.05 Q1.2
PWM-ILIM
  Bottom 0.61: R22.2 81.6,63.82 83.19,62.23 85.72,62.23 Q1.3
PWM-OUT
  Bottom 0.61: PWM.RING 91.68,54.05 90.49,55.24 90.49,60.01 Q1.1
PWRLED
  Bottom 0.813: R14.2 PWR.A
RA+/SO
  Top 0.203: JP1.1 21.11,1.11 47.78,1.11 53.02,6.35 53.02,7.3 55.24,9.53 59.05,9.53 61.12,7.46 61.12,5.4 65.56,0.95 73.5,0.95 76.04,3.49 JP2.1
  Bottom 0.61: IC1.32 29.21,24.13 27.62,22.54 27.62,21.59 23.81,17.78 23.81,7.3 23.18,6.67 21.59,6.67 18.73,3.81 JP1.1 | JP2.1 77.15,3.81 80.01,6.67 81.28,6.67 85.41,10.79 89.85,10.79 ST4.6
RA-1A  (via drill 0.8)
  Top 1.422: v84.45,20.95 v84.45,25.4
  Bottom 1.27: M2.12 v84.45,20.95
  Bottom 1.422: v84.45,25.4 RA.5
RA-1B
  Bottom 1.422: M2.11 77.79,18.73 87.31,18.73 RA.2
RA-2A
  Bottom 1.422: RA.3 87.31,23.18 83.19,23.18 82.87,23.5 M2.13
RA-2B
  Bottom 1.422: M2.14 81.92,26.04 83.5,27.62 88.9,27.62 90.17,26.35 RA.4
RA-/!SS
  Top 0.203: JP1.4 27.3,2.54 47.31,2.54 51.59,6.83 51.59,7.78 54.77,10.95 59.53,10.95 62.55,7.94 62.55,5.87 66.04,2.38 73.03,2.38 76.36,5.71 82.87,5.71 JP2.4
  Bottom 0.61: IC1.35 28.26,16.51 27.62,15.88 27.62,5.4 26.35,4.13 JP1.4 | ST4.3 87,6.67 85.09,4.76 JP2.4
RESET  (via drill 0.8 pad 1.52)
  Top 0.61: v37.15,23.18 v37.15,40.96
  Bottom 0.406: 31.75,40.64 27.94,40.64
  Bottom 0.61: 61.91,13.65 60.96,14.61 60.96,15.88 54.29,22.54 53.34,22.54 49.85,26.04 49.21,26.04 47.31,24.13 IC1.9 42.23,24.13 41.27,23.18 v37.15,23.18 | v37.15,40.96 36.83,40.64 31.75,40.64 | 27.94,40.64 25.72,38.42 C9.2 | R20.1 61.91,13.65 | 61.91,13.65 62.55,13.02 arc-16 64.14,11.43 65.41,11.43 67.31,13.34 73.34,13.34 75.56,11.11 75.56,8.57 75.88,8.26 75.88,6.99 73.34,4.45 PROG.5
RX  (via drill 0.8 pad 1.52)
  Top 0.61: v40.96,30.16 v40.96,44.77
  Bottom 0.406: 31.43,45.72 28.26,45.72
  Bottom 0.61: 31.43,45.72 40.01,45.72 v40.96,44.77 | 28.26,45.72 27.3,45.72 R16.1 | IC1.11 41.59,29.21 40.96,29.84 v40.96,30.16
RX(USB)
  Bottom 0.61: IC2.12 13.34,37.47 14.92,39.05 14.92,40.96 R16.2
STAT-SCLK
  Bottom 0.61: R13.1 12.7,1.27 31.14,1.27 37.47,7.6 | 37.47,7.6 37.47,15.56 43.5,21.59 IC1.8 | 37.47,7.6 40.96,4.1 40.96,2.86 42.55,1.27 50.16,1.27 53.02,4.13 53.02,6.03 arc-159 61.12,6.51 65.09,2.54 68.58,2.54 69.53,3.49 PROG.3
STATLED
  Bottom 1.016: STAT.A 4.76,4.49 R13.2
STEP-1
  Bottom 0.406: 43.5,43.18 46.67,43.18
  Bottom 0.61: IC1.29 35.56,31.75 42.23,38.42 42.23,41.91 43.5,43.18 | 46.67,43.18 47.31,42.55 47.31,41.91 51.12,38.1 51.75,38.1 53.66,36.2 60.01,36.2 61.28,37.47 63.5,37.47 M1.7
STEP-2  (via drill 0.8 pad 1.52)
  Top 0.61: v60.33,28.26 v60.33,21.27
  Bottom 0.61: IC1.14 46.67,36.83 49.21,34.29 49.85,34.29 51.75,32.38 53.02,32.38 56.52,28.89 57.47,28.89 57.78,28.57 60.01,28.57 v60.33,28.26 | v60.33,21.27 60.33,20.32 M2.7
TX  (via drill 0.8 pad 1.52)
  Top 0.61: v39.05,26.67 v39.05,42.86
  Bottom 0.406: 28.57,43.18 31.75,43.18
  Bottom 0.61: v39.05,26.67 IC1.10 | R15.1 27.3,43.18 28.57,43.18 | 31.75,43.18 38.73,43.18 v39.05,42.86
TX(USB)
  Bottom 0.61: IC2.10 20.32,41.27 R15.2
USBLED
  Bottom 0.61: USB.A 6.35,31.39 R19.1
USBOSC1
  Bottom 0.61: IC2.2 18.1,19.68 17.46,19.05 17.46,15.56 19.68,13.34 X2.1 22.23,12.38 C8.1
USBOSC2
  Bottom 0.61: IC2.3 18.1,22.23 16.19,20.32 X2.2 17.46,12.06 C7.1
USBSTAT
  Bottom 0.61: IC2.16 12.38,27.3 9.53,30.16 8.26,30.16 R19.2
V+  (via drill 0.8, 0.8 pad 1.52)
  Top 1.016: IC3.3 14.61,64.45 14.61,63.82 | v83.82,64.14 v83.82,53.34
  Top 1.778: 14.61,63.82 D1.C 14.61,64.14 28.57,64.14 29.21,64.77 52.39,64.77 52.39,60.52 arc180 61.59,60.52 61.59,64.77 71.75,64.77 v71.75,58.1 C2.+ 75.88,58.1 76.2,57.78 76.2,57.15 arc37 77.47,53.34 M1.16
  Bottom 0.61: C10.1 64.77,64.77 | D1.C 14.61,63.5 14.61,64.45 14.29,64.45
  Bottom 1.016: IC3.3 14.29,64.45 | v83.82,64.14 92.39,64.14 PWM.TIP | v83.82,53.34 77.47,53.34
  Bottom 1.778: v71.75,58.1 71.75,64.77 64.77,64.77 61.59,64.77 61.59,60.52 arc-180 52.39,60.52 52.39,64.77 29.21,64.77 28.57,64.14 14.61,64.14 14.61,63.5 | v71.75,58.1 C2.+ 75.88,58.1 76.2,57.78 arc45 77.47,53.34 M1.16 | v71.75,58.1 71.75,34.29 74.93,31.11 M2.16 80.01,31.11 C4.+
  pour Top (isolate 0.61): 3.17,66.04 3.17,61.28 6.99,61.28 6.99,54.93 36.2,54.93 36.2,56.83 arc-90 37.47,58.1 57.15,58.1 57.15,66.04
VBUS
  Bottom 1.016: USB->.VBUS 7.94,15.57 D2.A
VIN
  Top 1.93: J1.PWR 14.61,50.44 D1.A
  Bottom 1.93: J1.PWR 14.61,50.44 D1.A
VPIC
  Bottom 0.406: 11.11,26.04 14.61,26.04 | 18.73,23.5 21.91,23.5
  Bottom 0.61: 14.61,26.04 17.14,23.5 18.73,23.5 | 21.91,23.5 22.54,22.86 22.54,18.73 20.95,17.14 IC2.1 | 11.11,26.04 10.16,26.04 9.84,26.35 | D2.C 9.84,26.35 | 9.84,26.35 9.53,26.67 | 8.57,27.62 9.53,26.67 | 9.53,26.67 8.89,26.67 8.26,27.3
  Bottom 0.813: C5.1 5.08,26.04 5.4,26.35 D2.C 7.94,26.99 8.57,27.62 8.89,27.94 R18.2
VUSB
  Bottom 0.61: C6.2 5.71,24.13 9.21,24.13 9.84,24.77 IC2.17

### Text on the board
Bottom: Tom Carpenter | DEC | AstroEQ | V4.6-PTH | RA | 1 | ST4 | 1 | 1
tNames: AstroEQ | V4.6-PTH | Controller | Designed By | Tom Carpenter | (wire to / JP3) | (C) 2012-16 | 16M | 12V | 882x/4988 | IO1 (SNAP) | 8834 | (wire to JP4) | 1 | 8834 | +5V / IO0 / IO1 / IO2 / GND | 12M | 882x/4988 | ESTOP | 1 | 1 | IO3 / (SPEED)
tValues: 8824/5 | 8834 | 4988 | 8824/5 | 8834 | 4988 | Markings show the location of the Potentiometers on the | Pololu Boards depending on which chip they use.
Reference: This board design is for DIY/Kit AstroEQ boards | It is a 2 Layer board designed to be sent for manufacture. The AstroEQ-PTH-Gerber.zip file contains the required gerber files. | I use iteadstudio.com 10cm x 10cm prototype service, selecting 1.2mm thick, HASL, 100% electrical check

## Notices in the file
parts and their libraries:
SparkFun: Licensing: CC v3.0 Share-Alike You are welcome to use this library for commercial purposes.
